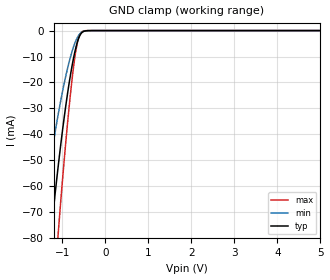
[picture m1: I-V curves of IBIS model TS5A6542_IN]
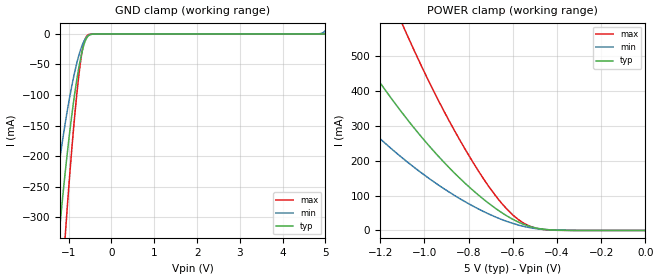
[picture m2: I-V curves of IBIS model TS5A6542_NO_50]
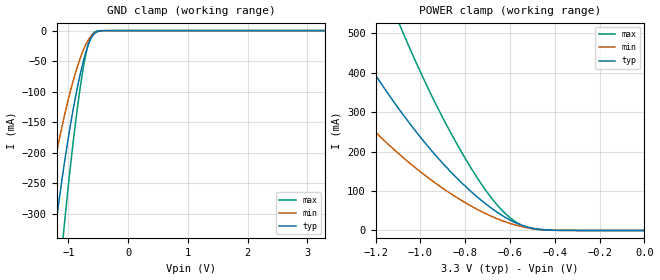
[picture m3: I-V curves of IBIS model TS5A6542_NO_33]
| TEXAS INSTRUMENTS INCORPORATED
| Standard Linear and Logic Group
| IBIS Model of TS5A6542
| 0.75-Ohm SPDT ANALOG SWITCH WITH INPUT LOGIC TRANSLATION
| This file contains package information for the following:
|  WLBGA 8-pin (YZP) package as [Component] TS5A6542_YZP
|  WLBGA 8-pin (YZT) package as [Component] TS5A6542_YZT
| This device can be powered at the following VPLUS values:
|  5 volt VPLUS
|  3.3 volt VPLUS
|  2.5 volt VPLUS
| This file provides unique models under the [Model Selector] for each VPLUS.
| For operation at a specific VPLUS, select the appropriate model after each
| [Model Selector] keyword.
| VIO is only powered to 1.8v, therefore no [Model Selector] is used for
| the input model.
[IBIS Ver]   3.2
[Comment char]  |_char
[File Name]   ts5a6542.ibs
[File Rev]   1.1 | x_die
[Date]   March 9, 2006
[Source]   Data created from TI-SPICE simulations at TI-SLL.
[Notes]   The following is an IBIS list for the TS5A6542.
   Please contact sllibis@ti.com with questions and
   comments concerning SLL IBIS models.
   - FILE REV HISTORY
   - 1.1 Release IBIS file on 05/19/06
   - Non-monotonic data due to FET characteristics.
   - NCH & PCH MOSFETS, so [Series Mosfet] model can have rising
   or falling currents
   - VIO is only powered to 1.8v, therefore no [Model Selector]
   is used for the input model.
[Disclaimer] Property of Texas Instruments Incorporated.  Unauthorized
   reproduction and/or distribution is strictly prohibited.
   This product is protected under copyright law.
   Created  2006, (C) Copyright  2006, Texas Instruments
   Incorporated, All Rights Reserved
   UNLESS THERE IS A SIGNED, WRITTEN AGREEMENT TO THE
   CONTRARY, TEXAS INSTRUMENTS (TI) IS PROVIDING THE IBIS
   MODELS  AND WITHOUT ANY WARRANTY, EXPRESSED OR
   IMPLIED.  TI assumes no liability for:
   1) the accuracy of the IBIS models provided to your
   company;
   2) the proper functioning of these IBIS Models in your
   design or for any resulting applications; or
   3) infringement of patents, copyrights or intellectual
   property rights resulting from your use of these IBIS
   models.
   TI provides IBIS Models as a service to our customers.
   You and your company shall not distribute, sell or give
   these models to anyone else without prior written
   permission from TI.
   TI reserves the right to make changes to our products or
   to discontinue any semiconductor product or service
   without notice, and advises our customers to obtain the
   latest version of relevant information to verify, before
   placing orders, that the information being relied on is
   current.
   Please be aware that your receipt and use of the IBIS
   information provided shall serve as acceptance of these
   terms and conditions.  If you do not accept these terms,
   you should return or destroy the IBIS models and any
   other accompanying information immediately.
| Component TS5A6542_YZP 8-PIN WLBGA
[Component]   TS5A6542_YZP
[Manufacturer]   Texas Instruments, Inc.
[Package]
|   typ   min   max
R_pkg   1.000e-03   1.000e-03   4.000e-03
L_pkg   6.400e-11   2.400e-11   3.790e-10
C_pkg   5.800e-14   0.000e+00   6.700e-14
[Pin]   signal_name   model_name   R_pin   L_pin   C_pin
1   NO   TS5A6542_NO   1.000e-03   2.500e-11   6.400e-14
2   GND   GND   1.000e-03   2.400e-11   6.700e-14
3   NC   TS5A6542_NO   1.000e-03   2.400e-11   6.700e-14
4   VIO   POWER   1.000e-03   2.500e-11   6.400e-14
5   VPLUS   POWER   1.000e-03   2.500e-11   6.400e-14
6   IN   TS5A6542_IN   1.000e-03   2.400e-11   6.700e-14
7   COM   TS5A6542_COM   1.000e-03   2.400e-11   6.700e-14
8   GND   GND   1.000e-03   2.500e-11   6.400e-14
| Component TS5A6542_YZT 8-PIN WLBGA
[Component]   TS5A6542_YZT
[Manufacturer]   Texas Instruments, Inc.
[Package]
|   typ   min   max
R_pkg   1.000e-03   1.000e-03   4.000e-03
L_pkg   6.400e-11   2.400e-11   3.790e-10
C_pkg   5.800e-14   0.000e+00   6.700e-14
[Pin]   signal_name   model_name   R_pin   L_pin   C_pin
1   NO   TS5A6542_NO   1.000e-03   2.500e-11   6.400e-14
2   GND   GND   1.000e-03   2.400e-11   6.700e-14
3   NC   TS5A6542_NO   1.000e-03   2.400e-11   6.700e-14
4   VIO   POWER   1.000e-03   2.500e-11   6.400e-14
5   VPLUS   POWER   1.000e-03   2.500e-11   6.400e-14
6   IN   TS5A6542_IN   1.000e-03   2.400e-11   6.700e-14
7   COM   TS5A6542_COM   1.000e-03   2.400e-11   6.700e-14
8   GND   GND   1.000e-03   2.500e-11   6.400e-14
[Series Switch Groups]
| Function Group States
On  1 /   | COM->NO IN HIGH
On  2 /   | COM->NC IN LOW
On  3 /   | NO->COM IN HIGH
On  4 /   | NC->COM IN LOW
[Series Pin Mapping]   pin_2   model_name   function_table_group
7   1   TS5A6542_COM_50_S   1
| 7   1   TS5A6542_COM_33_S   1
| 7   1   TS5A6542_COM_25A_S   1
7   3   TS5A6542_COM_50_S   2
| 7   3   TS5A6542_COM_33_S   2
| 7   3   TS5A6542_COM_25A_S   2
1   7   TS5A6542_NO_50_S   3
| 1   7   TS5A6542_NO_33_S   3
| 1   7   TS5A6542_NO_25A_S   3
3   7   TS5A6542_NO_50_S   4
| 3   7   TS5A6542_NO_33_S   4
| 3   7   TS5A6542_NO_25A_S   4
| Model TS5A6542_NO
[Model Selector]   TS5A6542_NO
TS5A6542_NO_50   5 volt VPLUS
TS5A6542_NO_33   3.3 volt VPLUS
TS5A6542_NO_25A   2.5 volt VPLUS
| Model TS5A6542_NO_S
[Model Selector]   TS5A6542_NO_S
TS5A6542_NO_50_S   5 volt VPLUS
TS5A6542_NO_33_S   3.3 volt VPLUS
TS5A6542_NO_25A_S   2.5 volt VPLUS
| Model TS5A6542_COM
[Model Selector]   TS5A6542_COM
TS5A6542_COM_50   5 volt VPLUS
TS5A6542_COM_33   3.3 volt VPLUS
TS5A6542_COM_25A   2.5 volt VPLUS
| Model TS5A6542_COM_S
[Model Selector]   TS5A6542_COM_S
TS5A6542_COM_50_S   5 volt VPLUS
TS5A6542_COM_33_S   3.3 volt VPLUS
TS5A6542_COM_25A_S   2.5 volt VPLUS
[Model]   TS5A6542_NO_50_S
Model_type  Series_switch
| variable   typ   min   max
C_comp   0   0   0
[Temperature Range]   40   100   -40
| Ambient temperature   25   85   -40
[Voltage range]   5   4.5   5.5
[On]
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[Off]
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[Model]   TS5A6542_NO_33_S
Model_type  Series_switch
| variable   typ   min   max
C_comp   0   0   0
[Temperature Range]   40   100   -40
| Ambient temperature   25   85   -40
[Voltage range]   3.3   3   3.6
[On]
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[Off]
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[Model]   TS5A6542_NO_25A_S
Model_type  Series_switch
| variable   typ   min   max
C_comp   0   0   0
[Temperature Range]   40   100   -40
| Ambient temperature   25   85   -40
[Voltage range]   2.5   2.25   2.75
[On]
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[Off]
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[Model]   TS5A6542_COM_50_S
Model_type  Series_switch
| variable   typ   min   max
C_comp   0   0   0
[Temperature Range]   40   100   -40
| Ambient temperature   25   85   -40
[Voltage range]   5   4.5   5.5
[On]
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[Off]
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[Model]   TS5A6542_COM_33_S
Model_type  Series_switch
| variable   typ   min   max
C_comp   0   0   0
[Temperature Range]   40   100   -40
| Ambient temperature   25   85   -40
[Voltage range]   3.3   3   3.6
[On]
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[Off]
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[Model]   TS5A6542_COM_25A_S
Model_type  Series_switch
| variable   typ   min   max
C_comp   0   0   0
[Temperature Range]   40   100   -40
| Ambient temperature   25   85   -40
[Voltage range]   2.5   2.25   2.75
[On]
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[Off]
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| Models and submodels in the file (13): TS5A6542_IN (Input), TS5A6542_NO_50_S (Series_switch), TS5A6542_NO_50 (Terminator), TS5A6542_NO_33_S (Series_switch), TS5A6542_NO_33 (Terminator), TS5A6542_NO_25A_S (Series_switch), TS5A6542_NO_25A (Terminator), TS5A6542_COM_50_S (Series_switch), TS5A6542_COM_50 (Terminator), TS5A6542_COM_33_S (Series_switch), TS5A6542_COM_33 (Terminator), TS5A6542_COM_25A_S (Series_switch), TS5A6542_COM_25A (Terminator)
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[Model]   TS5A6542_IN
Model_type  Input
Vinl=0.5775
Vinh=1.2675
| variable   typ   min   max
C_comp   3.06pF   2.67pF   3.50pF
[Temperature Range]   40   100   -40
| Ambient temperature   25   85   -40
[Voltage range]   5   4.5   5.5
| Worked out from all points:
|   GND clamp passes 1 mA (typ) near -0.55 V on its own axis
[GND Clamp]
| TS5A6542_IN
|   Voltage   I(typ)   I(min)   I(max)
-5V       -919.8mA   -692.3mA   -1.158A
-1.53V    -125.7mA   -81.04mA   -182.3mA
-1.48V    -116.5mA   -74.76mA   -169.7mA
-1.26V    -78.32mA   -49.24mA   -116.2mA
-1.1V     -53.56mA   -33.13mA   -80.11mA
-1.08V    -50.68mA   -31.28mA   -75.83mA
-905mV    -27.81mA   -16.79mA   -41.18mA
-810mV    -17.47mA   -10.39mA   -25mA
-730mV    -10.2mA    -6.007mA   -13.37mA
-625mV    -3.355mA   -2.083mA   -3.282mA
-510mV    -397.6uA   -322uA     -200.8uA
5V        319.6pA    1.086nA    45.57pA
[Model]   TS5A6542_NO_50
Model_type  Terminator
| variable   typ   min   max
C_comp   37.47pF   33.22pF   40.78pF
| C_tri-state   37.47pF   33.22pF   40.78pF
[Temperature Range]   40   100   -40
| Ambient temperature   25   85   -40
[Voltage range]   5   4.5   5.5
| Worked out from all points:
|   GND clamp passes 1 mA (typ) near -0.49 V on its own axis
|   POWER clamp passes 1 mA (typ) near -0.40 V on its own axis
[GND Clamp]
| TS5A6542_NO_50
|   Voltage   I(typ)   I(min)   I(max)
-5V       -4.853A    -3.618A    -6.311A
-1.44V    -504.9mA   -331.8mA   -742.4mA
-1.415V   -483.2mA   -317.1mA   -711mA
-1.245V   -344.1mA   -223.9mA   -507.3mA
-1.205V   -313.8mA   -203.7mA   -462.2mA
-1.085V   -228.8mA   -147.7mA   -334.7mA
-1.05V    -205.9mA   -132.7mA   -299.9mA
-910mV    -123.5mA   -79.01mA   -173.8mA
-755mV    -51.96mA   -33.16mA   -62.86mA
-650mV    -19mA      -12.82mA   -16.26mA
-530mV    -2.366mA   -2.218mA   -935uA
5V        3.284nA    5.736mA    99.34pA
[POWER Clamp]
| TS5A6542_NO_50
|   Voltage   I(typ)   I(min)   I(max)
-5V       6.643A     4.894A     9.428A
-1.66V    909.5mA    579.4mA    1.544A
-1.365V   581.9mA    364.5mA    1.01A
-1.1V     337.1mA    208.3mA    592.2mA
-1.075V   316.7mA    195.4mA    556.6mA
-915mV    198.1mA    121.3mA    346.7mA
-780mV    114.9mA    69.91mA    195.5mA
-665mV    57.56mA    35.22mA    89.29mA
-575mV    24.02mA    15.64mA    31.38mA
-525mV    11.87mA    8.35mA     12.86mA
-460mV    3.519mA    2.88mA     2.632mA
-84.45fV  3.284nA    19.44nA    144.1pA
[Model]   TS5A6542_NO_33
Model_type  Terminator
| variable   typ   min   max
C_comp   37.75pF   33.73pF   41.83pF
| C_tri-state   37.75pF   33.73pF   41.83pF
[Temperature Range]   40   100   -40
| Ambient temperature   25   85   -40
[Voltage range]   3.3   3   3.6
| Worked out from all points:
|   GND clamp passes 1 mA (typ) near -0.49 V on its own axis
|   POWER clamp passes 1 mA (typ) near -0.42 V on its own axis
[GND Clamp]
| TS5A6542_NO_33
|   Voltage   I(typ)   I(min)   I(max)
-3.3V     -2.616A    -1.871A    -3.539A
-1.445V   -508.6mA   -333.9mA   -748.4mA
-1.225V   -328.3mA   -213mA     -484.4mA
-1.085V   -228.4mA   -147.1mA   -334.5mA
-1.07V    -218.5mA   -140.6mA   -319.4mA
-910mV    -123.2mA   -78.56mA   -173.6mA
-775mV    -59.67mA   -37.84mA   -74.96mA
-720mV    -39.22mA   -25.04mA   -43.74mA
-665mV    -22.69mA   -14.94mA   -20.84mA
-560mV    -4.445mA   -3.7mA     -2.185mA
-385mV    -56.34uA   -94.69uA   -5.746uA
3.3V      1.967nA    70.1uA     64.78pA
[POWER Clamp]
| TS5A6542_NO_33
|   Voltage   I(typ)   I(min)   I(max)
-3.3V     3.327A     2.324A     5.02A
-1.59V    783.2mA    503.3mA    1.315A
-1.33V    512.5mA    325.6mA    872.2mA
-1.09V    303.8mA    191.5mA    518.5mA
-1.07V    288.4mA    181.7mA    491.9mA
-950mV    202.6mA    127.4mA    342.6mA
-810mV    117.9mA    74.09mA    192.8mA
-700mV    63.91mA    40.51mA    95.37mA
-600mV    26.47mA    17.89mA    32.44mA
-545mV    12.75mA    9.451mA    12.66mA
-465mV    2.871mA    2.635mA    1.751mA
-48.03fV  1.967nA    14.6nA     86.22pA
